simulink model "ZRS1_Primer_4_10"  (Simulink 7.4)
settings: Solver=ode45  StartTime=0.0  StopTime=10.0  FixedStep=1.e-5  MaxStep=0.01  RelTol=1.e-6
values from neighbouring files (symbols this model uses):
  kp = 18    [ZRS1_Primer4_10_1.m]    (also in ZRS1_Primer4_10_2.m; ZRS1_Primer4_10_nih_preiz.m = 30; ZRS1_Primer4_9.m = 19; ZRS2_primer_3_9_a.m = 5.95662143529)
  referenca = 1    [ZRS1_Primer4_10_1.m]    (also in ZRS1_Primer4_10_2.m; ZRS1_Primer4_10_nih_preiz.m; ZRS1_Primer4_9.m = 0)
  td = 0.351    [ZRS1_Primer4_10_1.m]    (also in ZRS1_Primer4_10_2.m = 0.7692; ZRS1_Primer4_10_nih_preiz.m = 0; ZRS1_Primer4_9.m = 0.210526315789)
  ti = 1.405    [ZRS1_Primer4_10_1.m]    (also in ZRS1_Primer4_10_2.m = 3.077; ZRS1_Primer4_10_nih_preiz.m = inf; ZRS1_Primer4_9.m = 2)

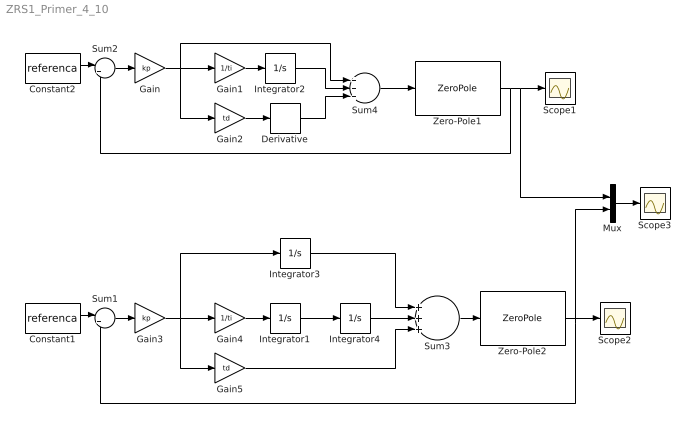
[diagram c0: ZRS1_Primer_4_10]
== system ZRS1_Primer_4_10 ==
  Constant1 : Constant  Value=referenca  OutDataType=sfix(16)  OutScaling=2^0
  Constant2 : Constant  Value=referenca  OutDataType=sfix(16)  OutScaling=2^0
  Derivative : Derivative
  Gain : Gain  Gain=kp  ParameterDataType=sfix(16)  ParameterScaling=2^0  OutDataType=sfix(16)  OutScaling=2^0
  Gain1 : Gain  Gain=1/ti  ParameterDataType=sfix(16)  ParameterScaling=2^0  OutDataType=sfix(16)  OutScaling=2^0
  Gain2 : Gain  Gain=td  ParameterDataType=sfix(16)  ParameterScaling=2^0  OutDataType=sfix(16)  OutScaling=2^0
  Gain3 : Gain  Gain=kp  ParameterDataType=sfix(16)  ParameterScaling=2^0  OutDataType=sfix(16)  OutScaling=2^0
  Gain4 : Gain  Gain=1/ti  ParameterDataType=sfix(16)  ParameterScaling=2^0  OutDataType=sfix(16)  OutScaling=2^0
  Gain5 : Gain  Gain=td  ParameterDataType=sfix(16)  ParameterScaling=2^0  OutDataType=sfix(16)  OutScaling=2^0
  Integrator{1..4} (4 alike) : Integrator
  Mux : Mux  Inputs=2
  Scope1 : Scope
  Scope2 : Scope
  Scope3 : Scope
  Sum1 : Sum  Inputs=|+-  OutDataType=sfix(16)  OutScaling=2^0
  Sum2 : Sum  Inputs=|+-  OutDataType=sfix(16)  OutScaling=2^0
  Sum3 : Sum  Inputs=+++  OutDataType=sfix(16)  OutScaling=2^0
  Sum4 : Sum  Inputs=+++  OutDataType=sfix(16)  OutScaling=2^0
  Zero-Pole1 : ZeroPole  Zeros=[]  Poles="[0 -1  -5]"  Gain=1
  Zero-Pole2 : ZeroPole  Zeros=[0]  Poles="[0 -1  -5]"  Gain=1
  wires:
  Constant2/1 -> Sum2/1
  Sum2/1 -> Gain/1
  Zero-Pole1/1 -> Sum2/2, Scope1/1, Mux/1
  Gain/1 -> Gain1/1, Sum4/1, Gain2/1
  Gain1/1 -> Integrator2/1
  Integrator2/1 -> Sum4/2
  Gain2/1 -> Derivative/1
  Derivative/1 -> Sum4/3
  Sum4/1 -> Zero-Pole1/1
  Constant1/1 -> Sum1/1
  Sum1/1 -> Gain3/1
  Zero-Pole2/1 -> Sum1/2, Scope2/1, Mux/2
  Gain3/1 -> Gain4/1, Gain5/1, Integrator3/1
  Gain4/1 -> Integrator1/1
  Sum3/1 -> Zero-Pole2/1
  Integrator1/1 -> Integrator4/1
  Gain5/1 -> Sum3/3
  Integrator4/1 -> Sum3/2
  Integrator3/1 -> Sum3/1
  Mux/1 -> Scope3/1
